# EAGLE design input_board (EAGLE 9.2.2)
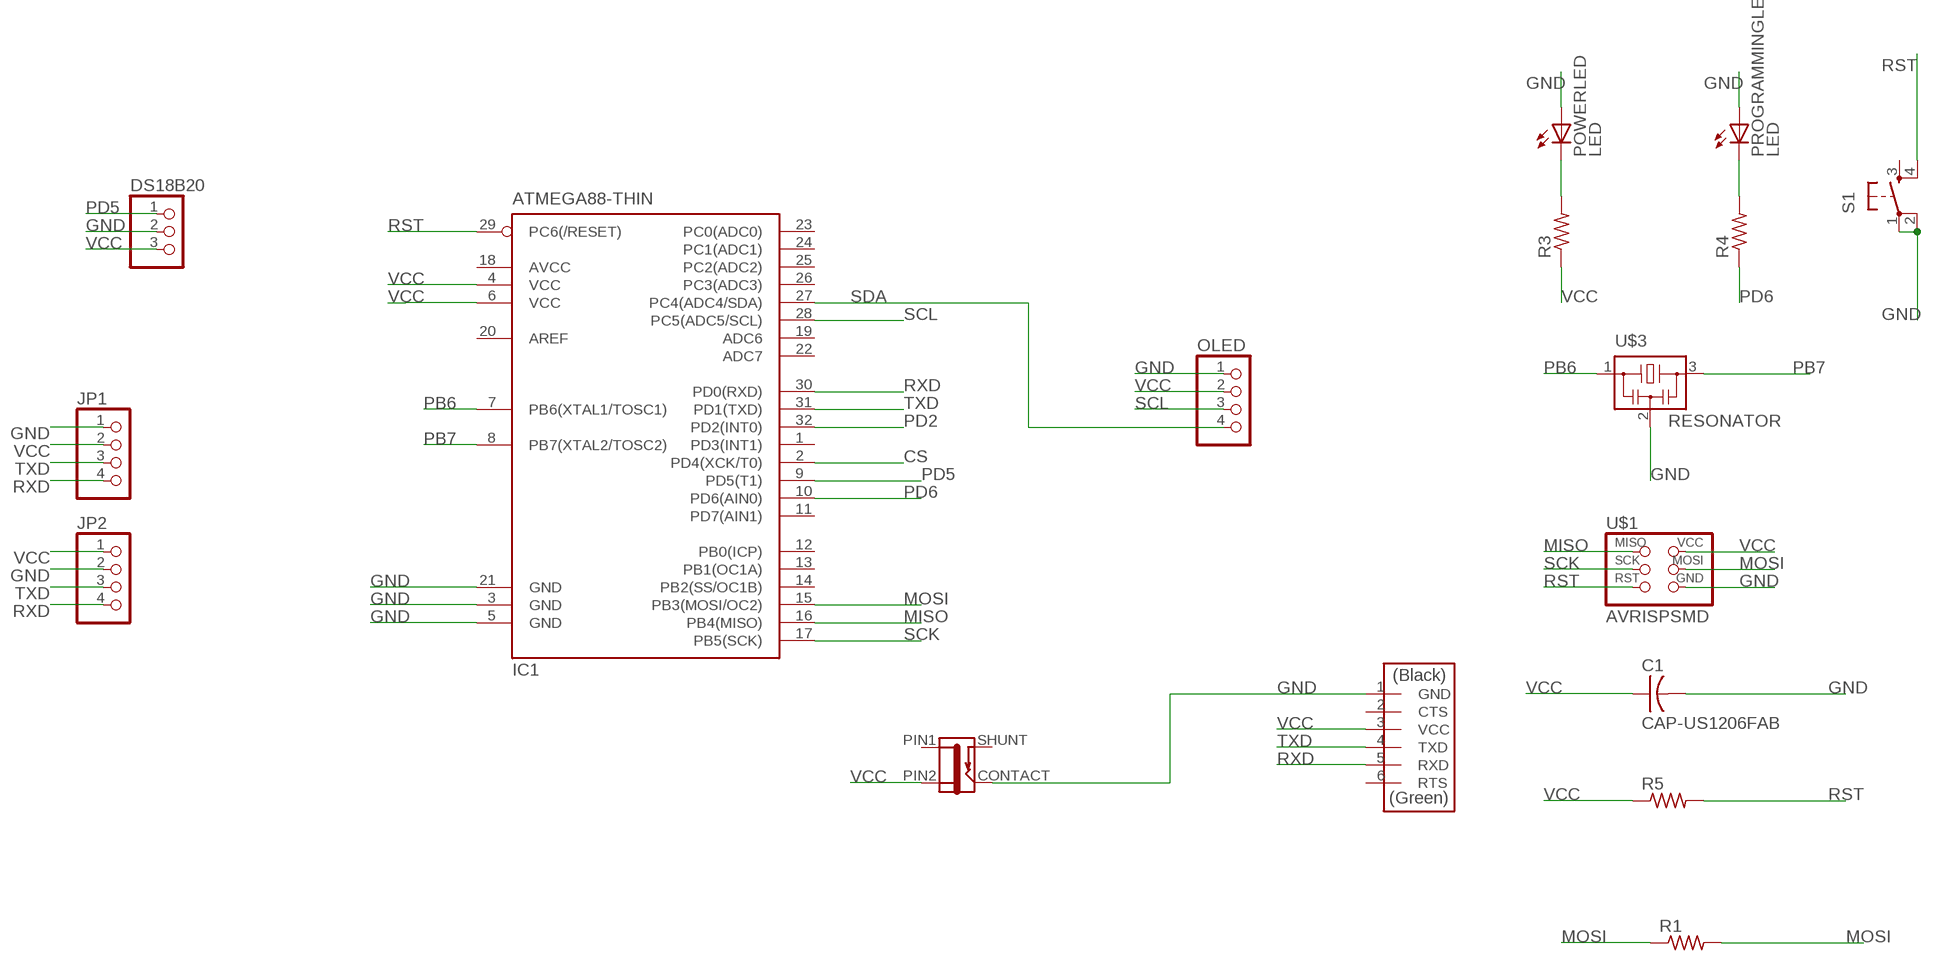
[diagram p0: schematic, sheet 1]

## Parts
C1  CAP-US1206FAB  [C1206FAB]
DS18B20  PINHD-1X3  [1X03]
FTDI  FTDI-SMD-HEADER  [1X06SMD]
IC1  ATMEGA88-THIN  [TQFP32-08THIN]
J1  JACK-2.1MM  [PJ-002AH-SMT]
JP1  PINHD-1X4  [1X04]
JP2  PINHD-1X4  [1X04]
OLED  PINHD-1X4  [1X04]
POWERLED  LED  [LED1206]
PROGRAMMINGLED  LED  [LED1206]
R1  RES-US1206FAB  [R1206FAB]
R3  RES-US1206FAB  [R1206FAB]
R4  RES-US1206FAB  [R1206FAB]
R5  RES-US1206FAB  [R1206FAB]
S1  6MM_SWITCH6MM_SWITCH  [6MM_SWITCH]
U$1  AVRISPSMD  [2X03SMD]
U$3  RESONATOR  [EFOBM]

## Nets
CS: IC1.2(PD4(XCK/T0))
GND: C1.2 DS18B20.2 FTDI.1(GND) IC1.3(GND) IC1.5(GND) IC1.21(GND) J1.CONTACT JP1.1 JP2.2 OLED.1 POWERLED.1(A) PROGRAMMINGLED.1(A) S1.1(P) S1.2(P1) U$1.6(GND) U$3.2
MISO: IC1.16(PB4(MISO)) U$1.1(MISO)
MOSI: IC1.15(PB3(MOSI/OC2)) R1.1 R1.2 U$1.4(MOSI)
N$6: POWERLED.2(C) R3.2
N$10: PROGRAMMINGLED.2(C) R4.2
PB6: IC1.7(PB6(XTAL1/TOSC1)) U$3.1
PB7: IC1.8(PB7(XTAL2/TOSC2)) U$3.3
PD2: IC1.32(PD2(INT0))
PD5: DS18B20.1 IC1.9(PD5(T1))
PD6: IC1.10(PD6(AIN0)) R4.1
RST: IC1.29(PC6(/RESET)) R5.2 S1.4(S1) U$1.5(RST)
RXD: FTDI.5(RXD) IC1.30(PD0(RXD)) JP1.4 JP2.4
SCK: IC1.17(PB5(SCK)) U$1.3(SCK)
SCL: IC1.28(PC5(ADC5/SCL)) OLED.3
SDA: IC1.27(PC4(ADC4/SDA)) OLED.4
TXD: FTDI.4(TXD) IC1.31(PD1(TXD)) JP1.3 JP2.3
VCC: C1.1 DS18B20.3 FTDI.3(VCC) IC1.4(VCC) IC1.6(VCC) J1.PIN2 JP1.2 JP2.1 OLED.2 R3.1 R5.1 U$1.2(VCC)
Unconnected: FTDI.2(CTS) FTDI.6(RTS) IC1.1(PD3(INT1)) IC1.11(PD7(AIN1)) IC1.12(PB0(ICP)) IC1.13(PB1(OC1A)) IC1.14(PB2(SS/OC1B)) IC1.19(ADC6) IC1.20(AREF) IC1.22(ADC7) IC1.23(PC0(ADC0)) IC1.24(PC1(ADC1)) IC1.25(PC2(ADC2)) IC1.26(PC3(ADC3)) S1.3(S)

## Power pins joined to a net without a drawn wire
AVCC: IC1.18(AVCC)
PIN1: J1.PIN1
SHUNT: J1.SHUNT

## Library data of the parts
C1 = fab:CAP-US
DS18B20 = pinhead:PINHD-1X3: PIN HEADER
FTDI = fab:FTDI-SMD-HEADER
IC1 = fab:ATMEGA88-THIN
J1 = fab:JACK-2.1MM: SMD DC power jack PJ-002AH-SMT As found in the fablab inventory. Made by Zaerc.
JP1 JP2 OLED = pinhead:PINHD-1X4: PIN HEADER
POWERLED PROGRAMMINGLED = fab:LED: LED
R1 R3-R5 = fab:RES-US: Resistor (US Symbol)
S1 = fab:6MM_SWITCH: OMRON SWITCH
U$1 = fab:AVRISP
U$3 = fab:RESONATOR

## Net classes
0 default: width 0.152 mm, clearance 0.4 mm

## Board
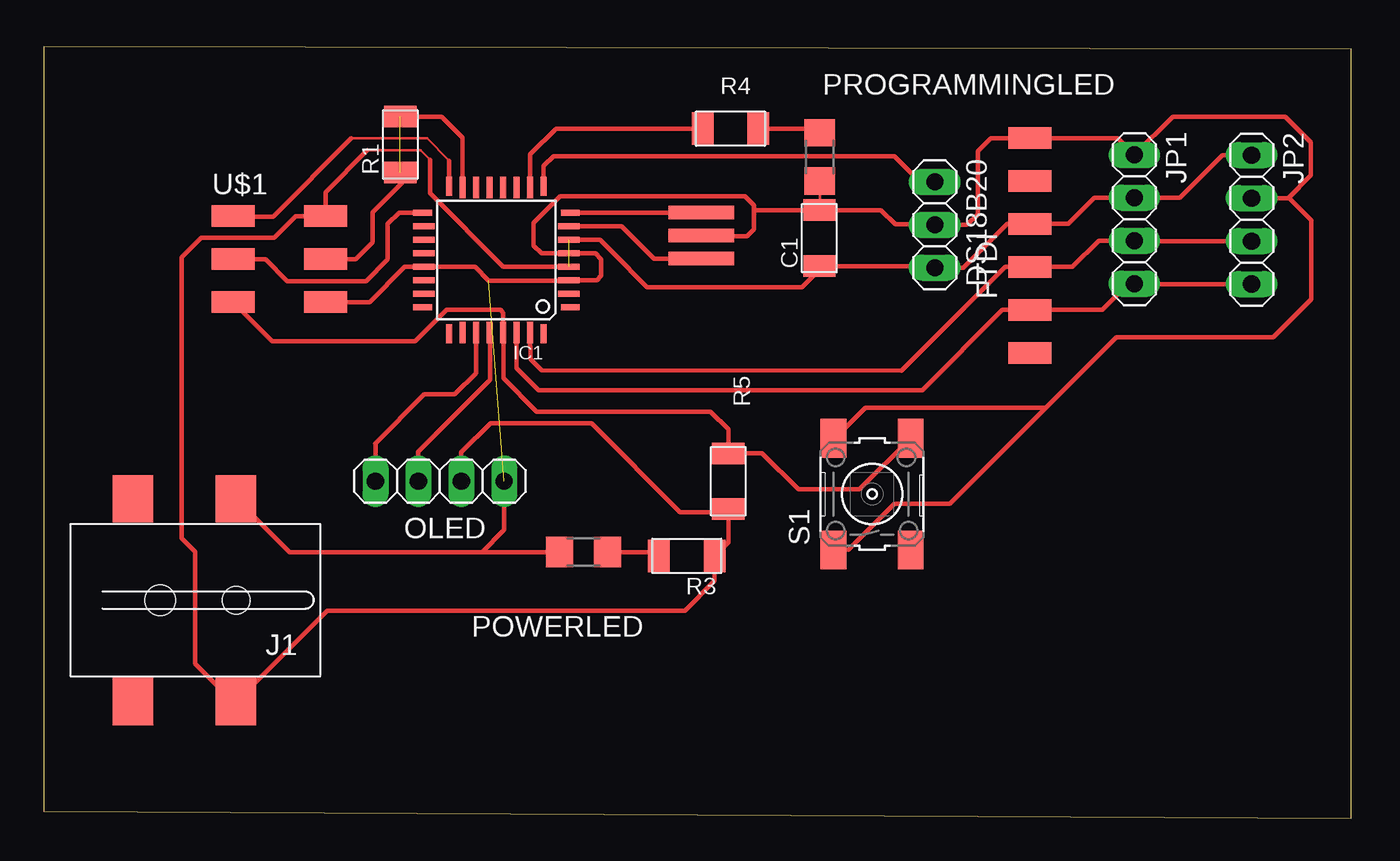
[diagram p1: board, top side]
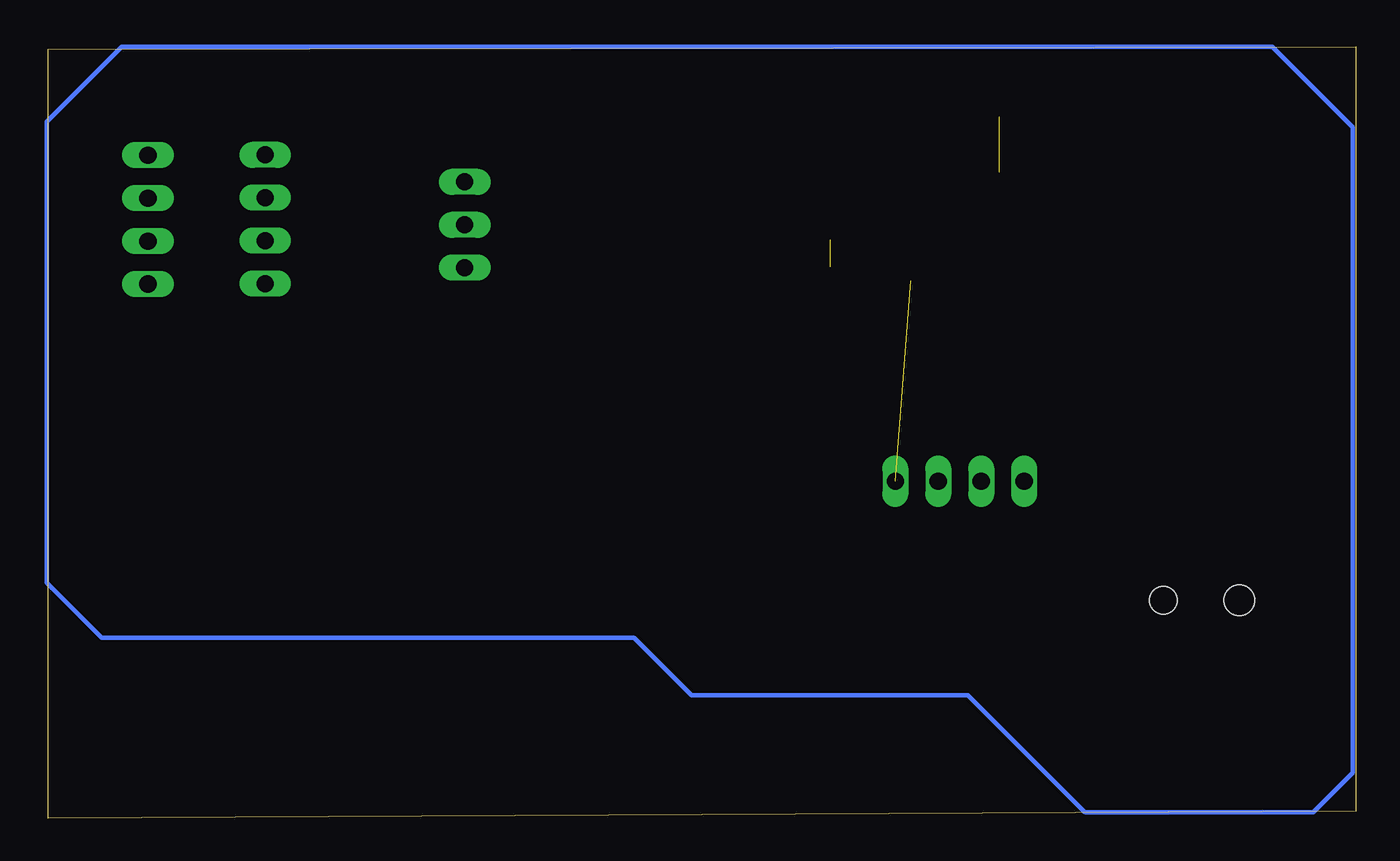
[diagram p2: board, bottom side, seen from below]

Size 77.37 x 45.62 mm. Coordinates in mm from the lower left corner, seen from the top.
Outline: 0,0.41 77.37,0 77.37,45.49 0.03,45.62 0,0.41
Copper layers (1*16): Top 0.035mm / dielectric 1.5mm / Bottom 0.035mm
Design rules "default *": minimum track width 6mil, minimum drill 0.35mm, track to track 0.4mm, track to pad 6mil, pad to pad 6mil, via to via 6mil, smd to smd 6mil, copper to edge 40mil, drill to drill 6mil, minimum pad ring 10mil, minimum via ring 8mil, stop-mask expansion 4mil, vias tented up to drill 0mil, thermal gap 10mil

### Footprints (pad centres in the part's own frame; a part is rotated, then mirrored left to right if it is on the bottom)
C1206FAB = smd 1.27 x 1.905: 1 -1.651,0; 2 1.651,0
1X03 = drill 1.016 long: 1 -2.54,0; 2 0,0; 3 2.54,0
1X06SMD = smd 2.54 x 1.27: 1 0,6.35; 2 0,3.81; 3 0,1.27; 4 0,-1.27; 5 0,-3.81; 6 0,-6.35
TQFP32-08THIN = smd 1.118 x 0.356: 1 -4.369,2.8; 8 -4.369,-2.8; 17 4.369,-2.8; 24 4.369,2.8 | smd 1.27 x 0.356: 2 -4.293,2; 3 -4.293,1.2; 4 -4.293,0.4; 5 -4.293,-0.4; 6 -4.293,-1.2; 7 -4.293,-2; 18 4.293,-2; 19 4.293,-1.2; 20 4.293,-0.4; 21 4.293,0.4; 22 4.293,1.2; 23 4.293,2 | smd 0.356 x 1.118: 9 -2.8,-4.369; 16 2.8,-4.369; 25 2.8,4.369; 32 -2.8,4.369 | smd 0.356 x 1.27: 10 -2,-4.293; 14 1.2,-4.293; 15 2,-4.293; 26 2,4.293; 27 1.2,4.293; 31 -2,4.293 | smd 0.35 x 1.27: 11 -1.2,-4.293; 12 -0.4,-4.293; 13 0.4,-4.293; 28 0.4,4.293; 29 -0.4,4.293; 30 -1.2,4.293
PJ-002AH-SMT = smd 2.4 x 2.8: CONTACT -2.4,-6; PIN1 3.7,6; PIN2 -2.4,6; SHUNT 3.7,-6 | hole 1.6: -2.4,0 | hole 1.8: 2.1,0
1X04 = drill 1.016 long: 1 -3.81,0; 2 -1.27,0; 3 1.27,0; 4 3.81,0
LED1206 = smd 1.6 x 1.803: 1 -1.422,0; 2 1.422,0
R1206FAB = smd 1.27 x 1.905: 1 -1.651,0; 2 1.651,0
6MM_SWITCH = smd 2.286 x 1.524: 1 -3.302,2.286; 2 3.302,2.286; 3 -3.302,-2.286; 4 3.302,-2.286
2X03SMD = smd 2.54 x 1.27: 1 -2.54,2.54; 2 2.92,2.54; 3 -2.54,0; 4 2.92,0; 5 -2.54,-2.54; 6 2.92,-2.54
EFOBM = smd 0.8 x 3.9: 1 -1.35,0; 2 0,0; 3 1.35,0

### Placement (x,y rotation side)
C1  45.9,34.32 90 top
DS18B20  52.73,35.1 270 top
FTDI  58.34,33.88 0 top
IC1  26.8,33.02 180 top
J1  8.99,12.9 180 top
JP1  64.54,35.43 270 top
JP2  71.48,35.41 270 top
OLED  23.44,19.94 180 top
POWERLED  31.95,15.75 0 top
PROGRAMMINGLED  45.92,39.12 90 top
R1  21.11,39.85 90 top
R3  38.05,15.52 180 top
R4  40.64,40.79 0 top
R5  40.51,19.94 90 top
S1  49.02,19.18 90 top
U$1  13.77,33.07 0 top
U$3  38.91,34.47 90 top

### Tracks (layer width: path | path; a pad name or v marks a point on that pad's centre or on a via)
CS
  Top 0.152: 31,30.98 IC1.2
GND  (1 unrouted)
  Top 0.152: 31,31.81 IC1.3 31.27,31.81 | 45.9,36.34 C1.2 46.23,35.97 45.92,36.27 PROGRAMMINGLED.1 | 38.96,34.42 U$3.2 | 52.7,35.13 DS18B20.2 | 11.74,18.97 11.46,18.97 J1.CONTACT | 22.49,32.63 IC1.21 22.54,32.58 22.73,32.58 22.7,32.61 | 47.62,15.87 S1.1
  Top 0.254: 31,31.81 26.34,31.81 25.53,32.61 22.7,32.61 21.36,32.61 19.28,30.53 U$1.6 | 42.04,35.97 42.04,36.25 41.5,36.78 30.55,36.78 29,35.23 29,33.86 29.45,33.41 IC1.5 32.64,33.42 32.99,33.07 32.99,32.08 32.73,31.82 IC1.3 | 42.04,35.97 42.04,34.85 41.6,34.42 38.96,34.42 | 42.04,35.97 C1.2 | 52.7,35.13 50.39,35.13 49.55,35.97 46.23,35.97 | DS18B20.2 54.63,35.1 55.27,35.74 55.27,39.45 56.06,40.23 FTDI.1 63.55,40.23 JP1.1 66.8,41.5 73.46,41.5 74.98,39.98 74.98,38.02 73.64,36.68 JP2.2 | 73.67,36.69 75.01,35.36 75.01,30.71 72.75,28.45 63.48,28.45 59.31,24.28 | S1.2 46.81,22.48 48.62,24.28 59.31,24.28 | 59.31,24.28 53.62,18.59 50.34,18.59 47.62,15.87 | J1.CONTACT 14.55,15.75 25.93,15.75 | 25.93,15.75 POWERLED.1 | OLED.1 27.25,17.07 25.93,15.75
MISO
  Top 0.152: IC1.16 | 11.09,35.53 11.16,35.58 U$1.1 | 24,38.89 22.68,40.21 18.21,40.21
  Top 0.254: 24,38.89 IC1.16 | 18.21,40.21 13.58,35.58 11.16,35.58
MOSI  (1 unrouted)
  Top 0.152: IC1.15 | 21.21,37.59 21.21,38.1 R1.1
  Top 0.254: R1.2 23.55,41.5 24.8,40.25 IC1.15 | U$1.4 18.47,33.07 19.46,34.06 19.46,35.84 21.21,37.59
N$1
  Bottom 0.254: 14.55,45.64 73.03,45.64 77.47,41.2 77.47,13.94 74.19,10.67 42.72,10.67 39.32,7.26 22.96,7.26 16.05,0.36 2.51,0.36 0.18,2.69 0.18,40.87 4.95,45.64 14.58,45.64
N$6
  Top 0.152: 36.17,15.75 R3.2
  Top 0.254: POWERLED.2 36.17,15.75
N$10
  Top 0.152: 45.67,40.79 PROGRAMMINGLED.2
  Top 0.254: R4.2 45.67,40.79
PB6
  Top 0.152: IC1.7 | 38.89,33.1 U$3.1
  Top 0.254: 38.89,33.1 36.12,33.1 34.2,35.02 IC1.7
PB7
  Top 0.152: IC1.8
  Top 0.254: IC1.8 U$3.3
PD5
  Top 0.152: 29.62,37.61 IC1.9 | 51.92,37.59 51.97,37.64 DS18B20.1
  Top 0.254: IC1.9 29.6,38.59 30.17,39.17 50.34,39.17 51.92,37.59
PD6
  Top 0.152: 28.79,37.33 IC1.10
  Top 0.254: IC1.10 28.8,39.26 30.33,40.79 R4.1
RST
  Top 0.152: IC1.29 | 11.48,30.28 U$1.5
  Top 0.254: IC1.29 27.21,26.02 29.17,24.05 39.47,24.05 40.51,23.01 R5.2 42.52,21.59 44.65,19.46 48.28,19.46 S1.4 | IC1.29 27.2,29.9 27.03,30.07 23.85,30.07 22,28.22 13.54,28.22 U$1.5
RXD
  Top 0.152: JP1.4 64.57,31.6 | 58.24,30.07 FTDI.5
  Top 0.254: IC1.30 27.99,26.62 29.29,25.32 51.99,25.32 56.74,30.07 58.24,30.07 | JP2.4 64.57,31.6 64.16,31.6 62.64,30.07 FTDI.5
SCK
  Top 0.152: 11.37,33.05 U$1.3
  Top 0.254: U$1.3 13.13,33.07 14.43,31.78 19.07,31.78 20.37,33.07 20.37,35.15 21.04,35.82 IC1.17
SCL
  Top 0.152: IC1.28
  Top 0.254: IC1.28 26.41,27.69 26.41,26.34 26.41,25.93 22.17,21.69 OLED.3
SDA
  Top 0.152: IC1.27 25.6,27.79 | 19.61,22.15 19.63,22.12
  Top 0.254: IC1.27 25.6,26.33 24.33,25.07 22.53,25.07 19.61,22.15 | 19.63,22.12 OLED.4
TXD
  Top 0.152: JP1.3 64.57,34.14
  Top 0.254: IC1.31 28.8,27.15 29.47,26.49 50.76,26.47 56.91,32.61 FTDI.4 60.88,32.61 62.43,34.16 JP1.3 | 64.57,34.14 JP2.3
VCC  (1 unrouted)
  Top 0.152: 31.27,32.63 IC1.4 | 45.81,32.48 C1.1 | 11.29,7.11 J1.PIN2 11.39,6.71 | 16.61,35.81 U$1.2 | 52.63,32.66 DS18B20.3 | 19.15,39.5 22.3,39.5 22.86,38.94 | 33.65,33.49 33.65,33.48 | 40.34,18.11 R5.1
  Top 0.254: 33.65,33.49 32.92,34.22 IC1.6 | 52.63,32.66 C1.1 45.9,32.44 44.88,31.42 35.71,31.42 33.65,33.48 | DS18B20.3 54.43,32.56 57.02,35.15 FTDI.3 60.63,35.15 62.18,36.7 JP1.2 67.23,36.7 69.75,39.22 JP2.1 | 19.15,39.5 16.69,37.03 U$1.2 14.91,35.61 13.63,34.33 9.34,34.33 8.18,33.17 8.18,16.56 8.97,15.77 8.97,9.13 11.39,6.71 | 22.86,38.94 22.86,36.96 27.19,32.63 31.27,32.63 | OLED.2 24.71,21.64 26.44,23.37 32.41,23.37 37.67,18.11 40.34,18.11 | R5.1 40.51,16.33 R3.1 39.7,14.05 37.94,12.29 16.78,12.29 J1.PIN2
